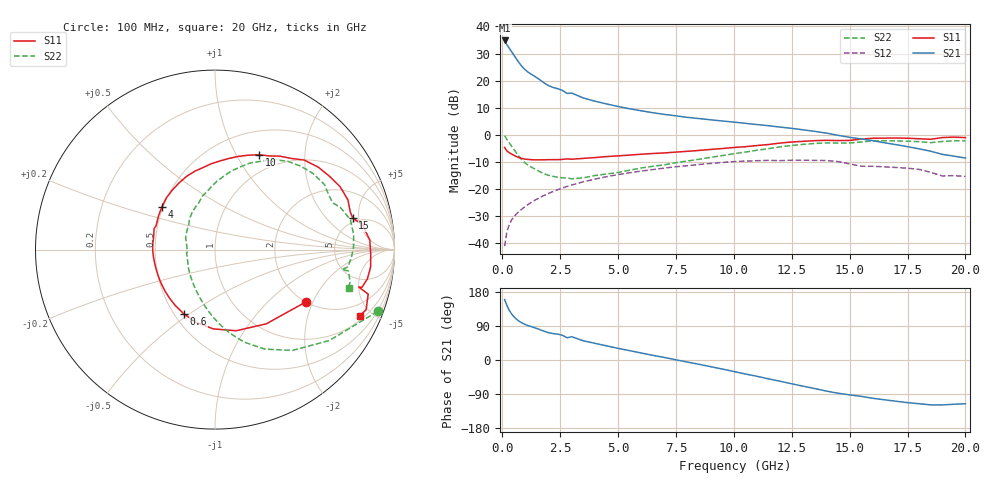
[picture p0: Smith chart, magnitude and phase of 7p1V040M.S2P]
! Infineon Technologies  Discrete & RF Semiconductors
! bfp620
! VCE =  1.0 V,  IC =  40 mA
! Common Emitter S-Parameters:  Sep 2002
# GHz  S  MA  R  50
!  f  S11  S21  S12  S22
! GHz  MAG  ANG  MAG  ANG  MAG  ANG  MAG  ANG
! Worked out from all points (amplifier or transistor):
!   59 points, 100 MHz to 20 GHz, reference 50 ohm
!   highest |S21| = 34.8 dB at 100 MHz (marker M1)
!   |S21| within 3 dB of that: start of sweep to 309.6 MHz
!   unconditionally stable (mu >= 1): 2.72 GHz to 2.897 GHz; 3.185 GHz to 9.975 GHz; 17.13 GHz to end of sweep
!   at 1 GHz: K = 0.83, MSG = 25.2 dB, |S12| = -26.4 dB
!   at 5.5 GHz: K = 1.04, MAG = 10.6 dB, |S12| = -14.0 dB
!   at 20 GHz: K = 1.39, MAG = -0.3 dB, |S12| = -15.4 dB
!   S11 on the Smith chart (normalised r, x): 100 MHz: 2.00, -1.77; 600 MHz: 0.56, -0.48; 4 GHz: 0.49, +0.28; 10 GHz: 0.78, +1.25; 15 GHz: 4.51, +4.13; 20 GHz: 1.24, -4.26
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0.1  0.5838 -30.0  55.13 159.5  0.0088 78.0  0.9693 -20.8
0.2  0.5028 -55.3  45.99 143.7  0.0163 68.8  0.814 -38.5
0.3  0.4672 -75.4  39.58 131.3  0.0221 64.8  0.7082 -52.5
0.4  0.4419 -91.2  34.26 121.7  0.0268 62.3  0.6194 -63.5
0.5  0.4189 -104.4  29.58 114.3  0.0307 60.7  0.5396 -72.6
0.6  0.3985 -115.6  25.51 108.4  0.0343 59.7  0.4692 -80.4
0.7  0.3821 -125.4  22.11 103.5  0.0377 59.1  0.4101 -87.3
0.8  0.37 -133.6  19.39 99.5  0.041 58.7  0.3628 -93.5
1  0.3555 -146.2  15.7 93.4  0.0478 58.5  0.2989 -103.9
1.2  0.3485 -155.1  13.54 89.0  0.0547 58.2  0.2613 -112.0
1.8  0.346 -176.0  9.131 76.1  0.0758 55.4  0.1922 -137.3
2.8  0.3589 161.0  5.796 58.7  0.1114 47.9  0.1597 -174.0
3  0.3541 158.1  5.887 61.4  0.1183 46.2  0.1544 -174.9
3.5  0.3672 148.8  4.781 50.6  0.1358 41.5  0.1605 170.4
4  0.3799 141.0  4.171 44.0  0.1522 36.7  0.1771 157.5
7  0.4631 97.8  2.382 6.7  0.243 6.6  0.2791 108.3
10  0.5829 65.1  1.717 -30.3  0.3205 -26.8  0.4476 78.2
10.5  0.6035 59.8  1.628 -37.0  0.328 -33.5  0.48 73.2
13.5  0.7802 26.7  1.156 -75.5  0.3372 -69.5  0.6922 37.7
15  0.7873 12.8  0.898 -92.0  0.29 -90.6  0.7057 21.7
17  0.8724 -6.4  0.659 -108.8  0.2495 -100.8  0.7722 1.1
20  0.8868 -24.5  0.373 -115.4  0.1708 -111.2  0.7743 -16.1
